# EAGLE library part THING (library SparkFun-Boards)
SparkFun Thing Board The SparkFun ESP8266 Thing is a breakout and development board for the ESP8266 WiFi SoC SparkFun Products: SparkFun ESP8266 Thing
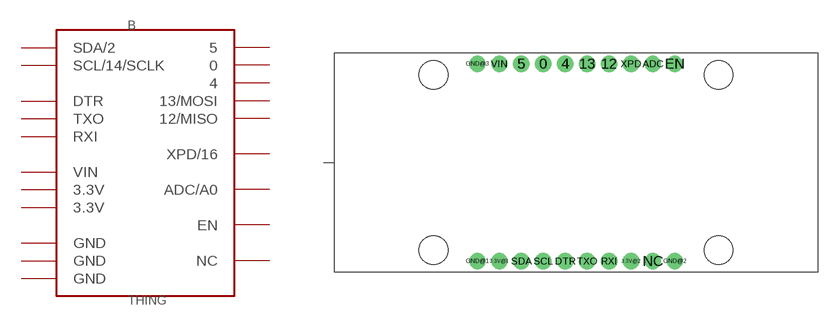
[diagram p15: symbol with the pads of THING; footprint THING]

Designator prefix B

## THING (SF_ID: WRL-13231)  [THING]
0  0
3.3V@1  3.3V  pwr
3.3V@2  3.3V  pwr
4  4
5  5
12  12/MISO
13  13/MOSI
ADC  ADC/A0
DTR  DTR
EN  EN  in
GND@1  GND  pwr
GND@2  GND  pwr
GND@3  GND  pwr
NC  NC  nc
RXI  RXI  in
SCL  SCL/14/SCLK
SDA  SDA/2
TXO  TXO  out
VIN  VIN  pwr
XPD  XPD/16

## Footprint THING (pad centres in mm)
SparkFun Thing Board Footprint Specifications: Pin count: 20 Pin pitch:0.1 inch Area: 2.2 x 1.0 inchees
drill 1.016 pad 1.88: 0 24.13,24.13; 3.3V@1 19.05,1.27; 3.3V@2 34.29,1.27; 4 26.67,24.13; 5 21.59,24.13; 12 31.75,24.13; 13 29.21,24.13; ADC 36.83,24.13; DTR 26.67,1.27; EN 39.37,24.13; GND@1 16.51,1.27; GND@2 39.37,1.27; GND@3 16.51,24.13; NC 36.83,1.27; RXI 31.75,1.27; SCL 24.13,1.27; SDA 21.59,1.27; TXO 29.21,1.27; VIN 19.05,24.13; XPD 34.29,24.13
hole 3.302 at 11.43,2.54
hole 3.302 at 11.43,22.86
hole 3.302 at 44.45,22.86
hole 3.302 at 44.45,2.54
